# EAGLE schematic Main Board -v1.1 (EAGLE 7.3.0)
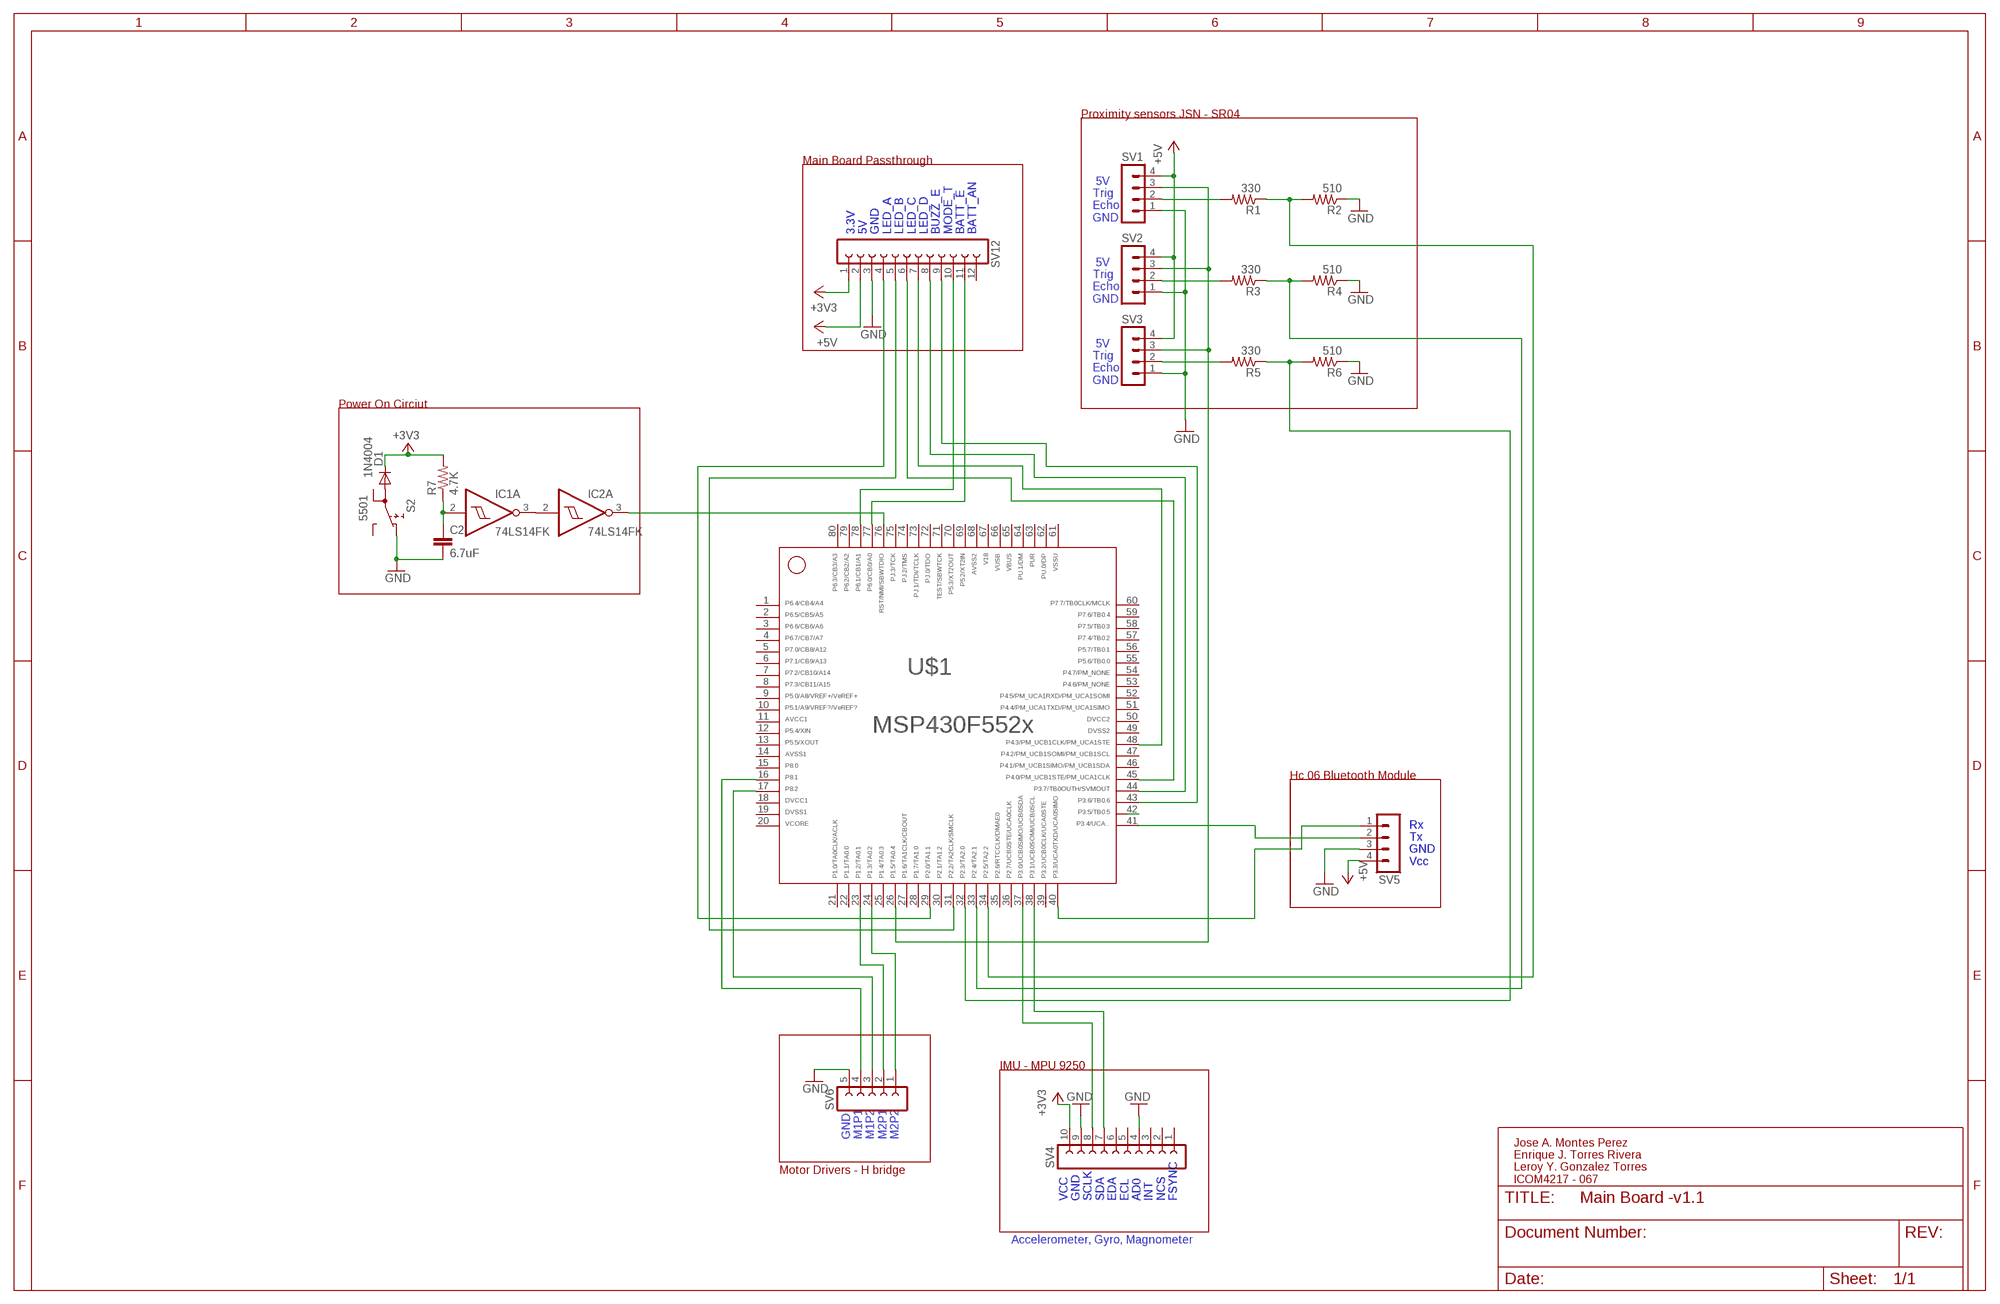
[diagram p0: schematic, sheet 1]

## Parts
C2  6.7uF  C2.5/6  [C2.5-6]
D1  1N4004  [DO41-10]
IC1  74LS14FK  [LCC20]
IC2  74LS14FK  [LCC20]
R1  330  R-US_0207/10  [0207/10]
R2  510  R-US_0207/10  [0207/10]
R3  330  R-US_0207/10  [0207/10]
R4  510  R-US_0207/10  [0207/10]
R5  330  R-US_0207/10  [0207/10]
R6  510  R-US_0207/10  [0207/10]
R7  4.7K  R-US_0207/7  [0207/7]
S2  5501  [5501]
SV1  MA04-1  [MA04-1]
SV2  MA04-1  [MA04-1]
SV3  MA04-1  [MA04-1]
SV4  FE10-1  [FE10]
SV5  MA04-1  [MA04-1]
SV6  FE05-1  [FE05-1]
SV12  FE12-1  [FE12]
U$1  F552X---PN80  [PN80]

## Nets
+3V3: D1.C R7.2 SV4.10 SV12.1
+5V: SV1.4 SV2.4 SV3.4 SV5.4 SV12.2
GND: C2.2 R2.1 R4.1 R6.1 S2.NC SV1.1 SV2.1 SV3.1 SV4.4 SV4.9 SV5.3 SV6.5 SV12.3
N$1: R1.2 SV1.2
N$2: D1.A S2.1A
N$3: IC1.3(A:O) IC2.2(A:I)
N$4: SV4.8 U$1.37
N$5: R1.1 R2.2 U$1.34
N$6: SV6.4 U$1.16
N$7: R3.2 SV2.2
N$8: SV6.3 U$1.17
N$9: SV12.10 U$1.78
N$10: SV6.2 U$1.23
N$11: SV6.1 U$1.24
N$12: R3.1 R4.2 U$1.33
N$13: SV12.11 U$1.77
N$14: SV4.7 U$1.38
N$15: SV5.1 U$1.40
N$16: IC2.3(A:O) U$1.76
N$17: R5.2 SV3.2
N$18: SV12.5 U$1.31
N$20: R5.1 R6.2 U$1.32
N$21: SV12.4 U$1.29
N$22: U$1.42
N$23: C2.1 IC1.2(A:I) R7.1
N$24: SV1.3 SV2.3 SV3.3 U$1.26
N$25: SV12.8 U$1.44
N$26: SV5.2 U$1.41
N$27: SV12.6 U$1.45
N$28: SV12.7 U$1.48
N$30: SV12.9 U$1.43
Unconnected: IC1.4(B:I) IC1.6(B:O) IC1.8(C:I) IC1.9(C:O) IC1.12(D:O) IC1.13(D:I) IC1.14(E:O) IC1.16(E:I) IC1.18(F:O) IC1.19(F:I) IC2.4(B:I) IC2.6(B:O) IC2.8(C:I) IC2.9(C:O) IC2.12(D:O) IC2.13(D:I) IC2.14(E:O) IC2.16(E:I) IC2.18(F:O) IC2.19(F:I) S2.1B S2.NO SV4.1 SV4.2 SV4.3 SV4.5 SV4.6 SV12.12 U$1.1 U$1.2 U$1.3 U$1.4 U$1.5 U$1.6 U$1.7 U$1.8 U$1.9 U$1.10 U$1.12 U$1.13 U$1.15 U$1.21 U$1.22 U$1.25 U$1.27 U$1.28 U$1.30 U$1.35 U$1.36 U$1.39 U$1.46 U$1.47 U$1.51 U$1.52 U$1.53 U$1.54 U$1.55 U$1.56 U$1.57 U$1.58 U$1.59 U$1.60 U$1.62 U$1.63 U$1.64 U$1.69 U$1.70 U$1.71 U$1.72 U$1.73 U$1.74 U$1.75 U$1.79 U$1.80

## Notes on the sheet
- Proximity sensors JSN - SR04
- Main Board Passthrough
- 5V
  Trig
  Echo
  GND
- 3.3V
  5V
  GND
  LED_A
  LED_B
  LED_C
  LED_D
  BUZZ_E
  MODE_T
  BATT_E
  BATT_AN
- 5V
  Trig
  Echo
  GND
- 5V
  Trig
  Echo
  GND
- Power On Circiut
- Hc 06 Bluetooth Module
- Rx
  Tx
  GND
  Vcc
- IMU - MPU 9250
- GND
  M1P1
  M1P2
  M2P1
  M2P2
- Motor Drivers - H bridge
- Jose A. Montes Perez
  Enrique J. Torres Rivera
  Leroy Y. Gonzalez Torres
  ICOM4217 - 067
- VCC
  GND
  SCLK
  SDA
  EDA
  ECL
  AD0
  INT
  NCS
  FSYNC
- Accelerometer, Gyro, Magnometer

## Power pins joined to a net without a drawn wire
11: U$1.11
14: U$1.14
18: U$1.18
19: U$1.19
20: U$1.20
49: U$1.49
50: U$1.50
61: U$1.61
65: U$1.65
66: U$1.66
67: U$1.67
68: U$1.68
GND: IC1.10(P:GND) IC2.10(P:GND)
VCC: IC1.20(P:VCC) IC2.20(P:VCC)

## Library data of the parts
C2 = capacitor-wima:C: CAPACITOR
D1 = diode:1N4004: DIODE
IC1 IC2 = 74xx-eu:74*14: Hex schmitt trigger INVERTER
R1-R6 = resistor:R-US_: RESISTOR, American symbol
R7 = rcl:R-US_: RESISTOR, American symbol
S2 = switch:55?: PUSHBUTTON SERIES 5500 SWITCHES Source: www.e-switch.com .. 5500.pdf
SV1-SV3 SV5 = con-lstb:MA04-1: PIN HEADER; OC_FARNELL: unknown; OC_NEWARK: unknown
SV4 = con-lsta:FE10-1: FEMALE HEADER; OC_FARNELL: unknown; OC_NEWARK: unknown
SV6 = con-lsta:FE05-1: FEMALE HEADER; OC_FARNELL: unknown; OC_NEWARK: unknown
SV12 = con-lsta:FE12-1: FEMALE HEADER; OC_FARNELL: unknown; OC_NEWARK: unknown
U$1 = TI_MSP430_v16:F552X---PN80: ***MSP430F552X***PN80 http://www.ti.com/lit/gpn/msp430f5529 Rev1.0 06/2010 For F552X where X is 1,5,7,9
